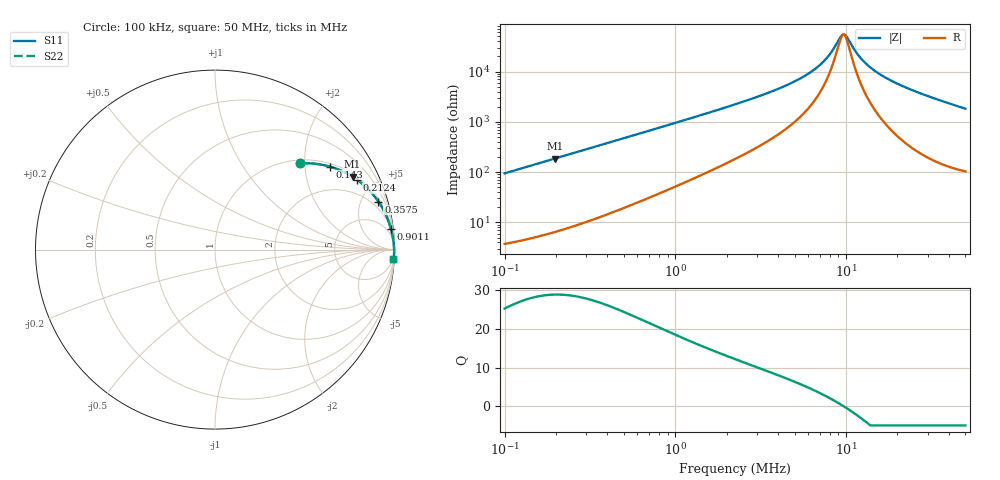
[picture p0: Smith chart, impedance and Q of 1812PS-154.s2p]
# MHz S MA R 50
!Freq  MagS11  AngS11  MagS21  AngS21  MagS12  AngS12  MagS22  AngS22
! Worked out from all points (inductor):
!   801 points, 100 kHz to 50 MHz, reference 50 ohm
!   read as one part in series: L = 150 uH near 103.2 kHz
!   highest Q = 28.9 at 196.6 kHz (marker M1), where L = 150 uH
!   self-resonance near 9.633 MHz
!   S11 on the Smith chart (normalised r, x): 100 kHz: 1.07, +1.88; 143 kHz: 1.10, +2.69; 212.4 kHz: 1.14, +4.00; 357.5 kHz: 1.25, +6.74; 901.1 kHz: 2, +17; 50 MHz: 3, -36
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0.1  0.6729 45.5  0.7136 -42.3  0.7136 -42.3  0.6729 45.5
0.1429522  0.7898 35.8  0.5859 -52.1  0.5859 -52.1  0.7898 35.8
0.1965681  0.8676 27.9  0.4681 -60.1  0.4681 -60.1  0.8676 27.9
0.2124468  0.8826 26.1  0.4406 -61.9  0.4406 -61.9  0.8826 26.1
0.2831897  0.9258 20.3  0.3466 -67.7  0.3466 -67.7  0.9258 20.3
0.3575105  0.9492 16.3  0.2814 -71.5  0.2814 -71.5  0.9492 16.3
0.7957584  0.9851 7.5  0.1306 -79.7  0.1306 -79.7  0.9851 7.5
0.9010744  0.9874 6.6  0.1154 -80.4  0.1154 -80.4  0.9874 6.6
2.236068  0.9953 2.6  0.04484 -82.7  0.04484 -82.7  0.9953 2.6
4.260918  0.9971 1.1  0.02017 -81.3  0.02017 -81.3  0.9971 1.1
6.332315  0.9978 0.5  0.009781 -76.5  0.009781 -76.5  0.9978 0.5
7.630124  0.998 0.3  0.005594 -68.6  0.005594 -68.6  0.998 0.3
8.310792  0.9981 0.2  0.003838 -59.4  0.003838 -59.4  0.9981 0.2
9.265618  0.9981 0.1  0.002072 -26.1  0.002072 -26.1  0.9981 0.1
9.707707  0.9982 -0.0  0.001829 3.4  0.001829 3.4  0.9982 -0.0
10.09219  0.9982 -0.1  0.00204 28.1  0.00204 28.1  0.9982 -0.1
11.51697  0.9983 -0.2  0.004241 65.9  0.004241 65.9  0.9983 -0.2
12.84016  0.9983 -0.4  0.006542 74.9  0.006542 74.9  0.9983 -0.4
14.76717  0.9983 -0.5  0.009724 79.9  0.009724 79.9  0.9983 -0.5
17.7937  0.9983 -0.8  0.01433 82.9  0.01433 82.9  0.9983 -0.8
27.06741  0.9979 -1.5  0.02685 84.8  0.02685 84.8  0.9979 -1.5
50  0.9954 -3.1  0.05448 83.6  0.05448 83.6  0.9954 -3.1
